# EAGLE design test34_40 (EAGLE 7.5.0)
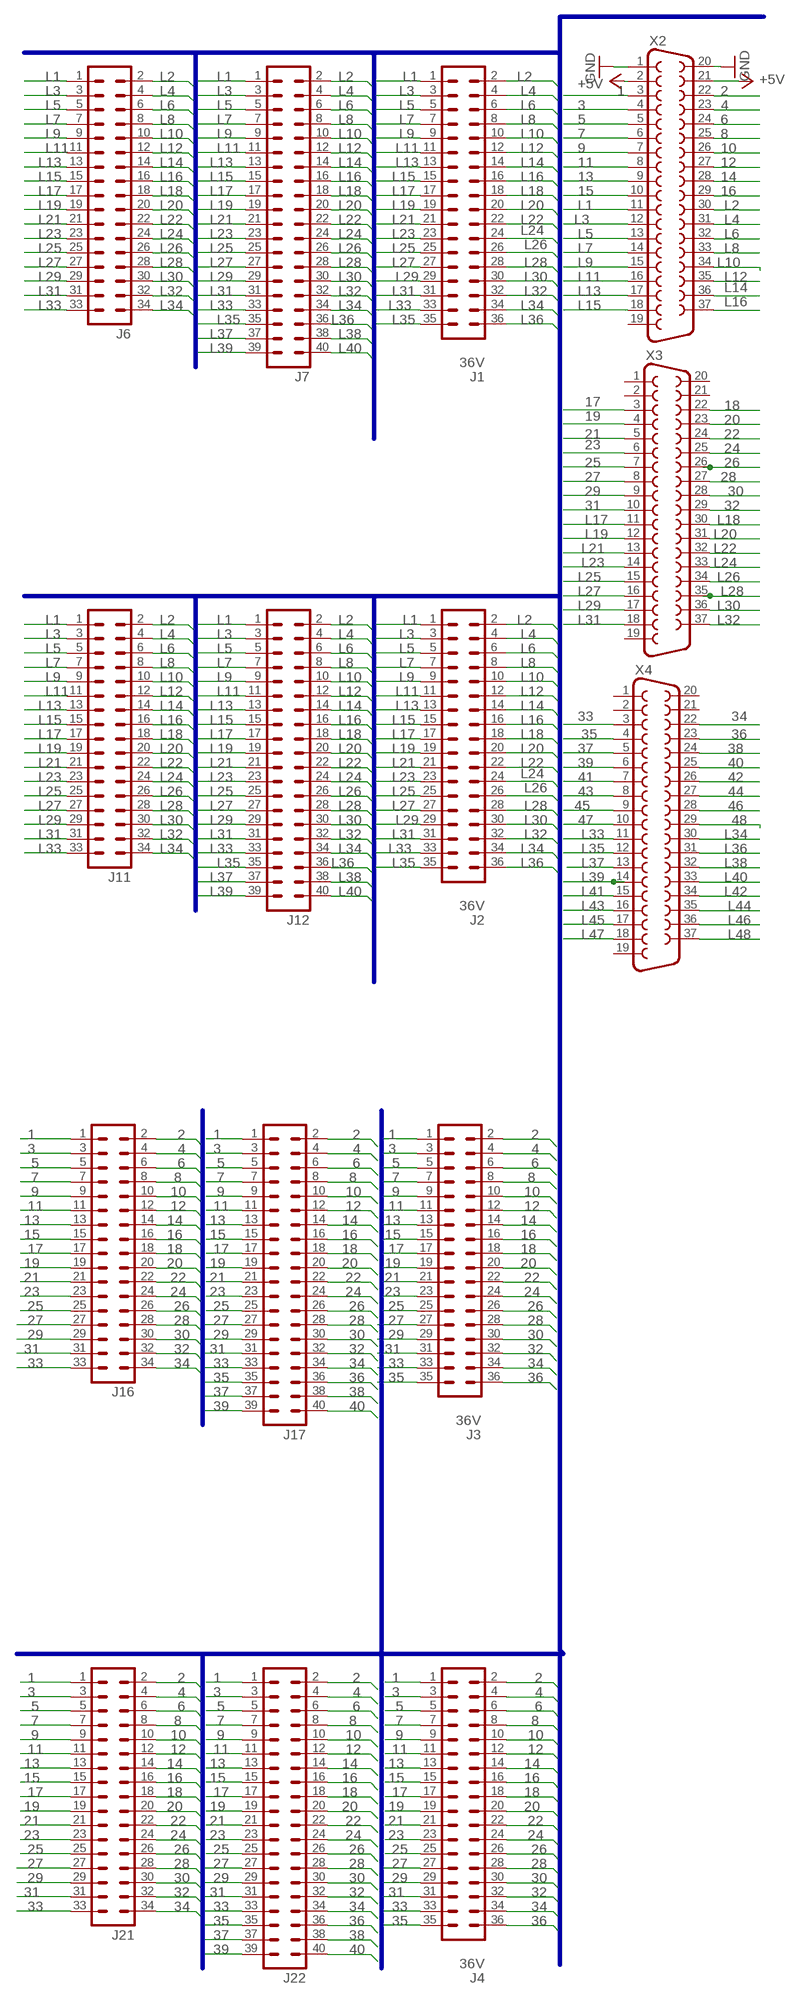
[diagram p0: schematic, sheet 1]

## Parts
J1  36V  [36V]
J2  36V  [36V]
J3  36V  [36V]
J4  36V  [36V]
J6  34V  [34V]
J7  40V  [40V]
J11  34V  [34V]
J12  40V  [40V]
J16  34V  [34V]
J17  40V  [40V]
J21  34V  [34V]
J22  40V  [40V]
X2  F37V  [F37V]
X3  F37V  [F37V]
X4  F37V  [F37V]

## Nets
1: J3.1 J4.1 J16.1 J17.1 J21.1 J22.1 X2.3
2: J3.2 J4.2 J16.2 J17.2 J21.2 J22.2 X2.22
3: J3.3 J4.3 J16.3 J17.3 J21.3 J22.3 X2.4
4: J3.4 J4.4 J16.4 J17.4 J21.4 J22.4 X2.23
5: J3.5 J4.5 J16.5 J17.5 J21.5 J22.5 X2.5
6: J3.6 J4.6 J16.6 J17.6 J21.6 J22.6 X2.24
7: J3.7 J4.7 J16.7 J17.7 J21.7 J22.7 X2.6
8: J3.8 J4.8 J16.8 J17.8 J21.8 J22.8 X2.25
9: J3.9 J4.9 J16.9 J17.9 J21.9 J22.9 X2.7
10: J3.10 J4.10 J16.10 J17.10 J21.10 J22.10 X2.26
11: J3.11 J4.11 J16.11 J17.11 J21.11 J22.11 X2.8
12: J3.12 J4.12 J16.12 J17.12 J21.12 J22.12 X2.27
13: J3.13 J4.13 J16.13 J17.13 J21.13 J22.13 X2.9
14: J3.14 J4.14 J16.14 J17.14 J21.14 J22.14 X2.28
15: J3.15 J4.15 J16.15 J17.15 J21.15 J22.15 X2.10
16: J3.16 J4.16 J16.16 J17.16 J21.16 J22.16 X2.29
17: J3.17 J4.17 J16.17 J17.17 J21.17 J22.17 X3.3
18: J3.18 J4.18 J16.18 J17.18 J21.18 J22.18 X3.22
19: J3.19 J4.19 J16.19 J17.19 J21.19 J22.19 X3.4
20: J3.20 J4.20 J16.20 J17.20 J21.20 J22.20 X3.23
21: J3.21 J4.21 J16.21 J17.21 J21.21 J22.21 X3.5
22: J3.22 J4.22 J16.22 J17.22 J21.22 J22.22 X3.24
23: J3.23 J4.23 J16.23 J17.23 J21.23 J22.23 X3.6
24: J3.24 J4.24 J16.24 J17.24 J21.24 J22.24 X3.25
25: J3.25 J4.25 J16.25 J17.25 J21.25 J22.25 X3.7
26: J3.26 J4.26 J16.26 J17.26 J21.26 J22.26 X3.26
27: J3.27 J4.27 J16.27 J17.27 J21.27 J22.27 X3.8
28: J3.28 J4.28 J16.28 J17.28 J21.28 J22.28 X3.27
29: J3.29 J4.29 J16.29 J17.29 J21.29 J22.29 X3.9
30: J3.30 J4.30 J16.30 J17.30 J21.30 J22.30 X3.28
31: J3.31 J4.31 J16.31 J17.31 J21.31 J22.31 X3.10
32: J3.32 J4.32 J16.32 J17.32 J21.32 J22.32 X3.29
33: J3.33 J4.33 J16.33 J17.33 J21.33 J22.33 X4.3
34: J3.34 J4.34 J16.34 J17.34 J21.34 J22.34 X4.22
35: J3.35 J4.35 J17.35 J22.35 X4.4
36: J3.36 J4.36 J17.36 J22.36 X4.23
37: J17.37 J22.37 X4.5
38: J17.38 J22.38 X4.24
39: J17.39 J22.39 X4.6
40: J17.40 J22.40 X4.25
41: X4.7
42: X4.26
43: X4.8
44: X4.27
45: X4.9
46: X4.28
47: X4.10
48: X4.29
+5V: X2.2 X2.21
GND: X2.1 X2.20
L1: J1.1 J2.1 J6.1 J7.1 J11.1 J12.1 X2.11
L2: J1.2 J2.2 J6.2 J7.2 J11.2 J12.2 X2.30
L3: J1.3 J2.3 J6.3 J7.3 J11.3 J12.3 X2.12
L4: J1.4 J2.4 J6.4 J7.4 J11.4 J12.4 X2.31
L5: J1.5 J2.5 J6.5 J7.5 J11.5 J12.5 X2.13
L6: J1.6 J2.6 J6.6 J7.6 J11.6 J12.6 X2.32
L7: J1.7 J2.7 J6.7 J7.7 J11.7 J12.7 X2.14
L8: J1.8 J2.8 J6.8 J7.8 J11.8 J12.8 X2.33
L9: J1.9 J2.9 J6.9 J7.9 J11.9 J12.9 X2.15
L10: J1.10 J2.10 J6.10 J7.10 J11.10 J12.10 X2.34
L11: J1.11 J2.11 J6.11 J7.11 J11.11 J12.11 X2.16
L12: J1.12 J2.12 J6.12 J7.12 J11.12 J12.12 X2.35
L13: J1.13 J2.13 J6.13 J7.13 J11.13 J12.13 X2.17
L14: J1.14 J2.14 J6.14 J7.14 J11.14 J12.14 X2.36
L15: J1.15 J2.15 J6.15 J7.15 J11.15 J12.15 X2.18
L16: J1.16 J2.16 J6.16 J7.16 J11.16 J12.16 X2.37
L17: J1.17 J2.17 J6.17 J7.17 J11.17 J12.17 X3.11
L18: J1.18 J2.18 J6.18 J7.18 J11.18 J12.18 X3.30
L19: J1.19 J2.19 J6.19 J7.19 J11.19 J12.19 X3.12
L20: J1.20 J2.20 J6.20 J7.20 J11.20 J12.20 X3.31
L21: J1.21 J2.21 J6.21 J7.21 J11.21 J12.21 X3.13
L22: J1.22 J2.22 J6.22 J7.22 J11.22 J12.22 X3.32
L23: J1.23 J2.23 J6.23 J7.23 J11.23 J12.23 X3.14
L24: J1.24 J2.24 J6.24 J7.24 J11.24 J12.24 X3.33
L25: J1.25 J2.25 J6.25 J7.25 J11.25 J12.25 X3.15
L26: J1.26 J2.26 J6.26 J7.26 J11.26 J12.26 X3.34
L27: J1.27 J2.27 J6.27 J7.27 J11.27 J12.27 X3.16
L28: J1.28 J2.28 J6.28 J7.28 J11.28 J12.28 X3.35
L29: J1.29 J2.29 J6.29 J7.29 J11.29 J12.29 X3.17
L30: J1.30 J2.30 J6.30 J7.30 J11.30 J12.30 X3.36
L31: J1.31 J2.31 J6.31 J7.31 J11.31 J12.31 X3.18
L32: J1.32 J2.32 J6.32 J7.32 J11.32 J12.32 X3.37
L33: J1.33 J2.33 J6.33 J7.33 J11.33 J12.33 X4.11
L34: J1.34 J2.34 J6.34 J7.34 J11.34 J12.34 X4.30
L35: J1.35 J2.35 J7.35 J12.35 X4.12
L36: J1.36 J2.36 J7.36 J12.36 X4.31
L37: J7.37 J12.37 X4.13
L38: J7.38 J12.38 X4.32
L39: J7.39 J12.39 X4.14
L40: J7.40 J12.40 X4.33
L41: X4.15
L42: X4.34
L43: X4.16
L44: X4.35
L45: X4.17
L46: X4.36
L47: X4.18
L48: X4.37
Unconnected: X2.19 X3.1 X3.2 X3.19 X3.20 X3.21 X4.1 X4.2 X4.19 X4.20 X4.21

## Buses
B$1

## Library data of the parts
J1-J4 = con-harting-v:36V
J6 J11 J16 J21 = con-harting-v:34V: CONNECTOR; OC_FARNELL: unknown; OC_NEWARK: unknown
J7 J12 J17 J22 = con-harting-v:40V: CONNECTOR; OC_FARNELL: unknown; OC_NEWARK: unknown
X2-X4 = con-subd:F37: SUB-D; OC_FARNELL: unknown; OC_NEWARK: unknown

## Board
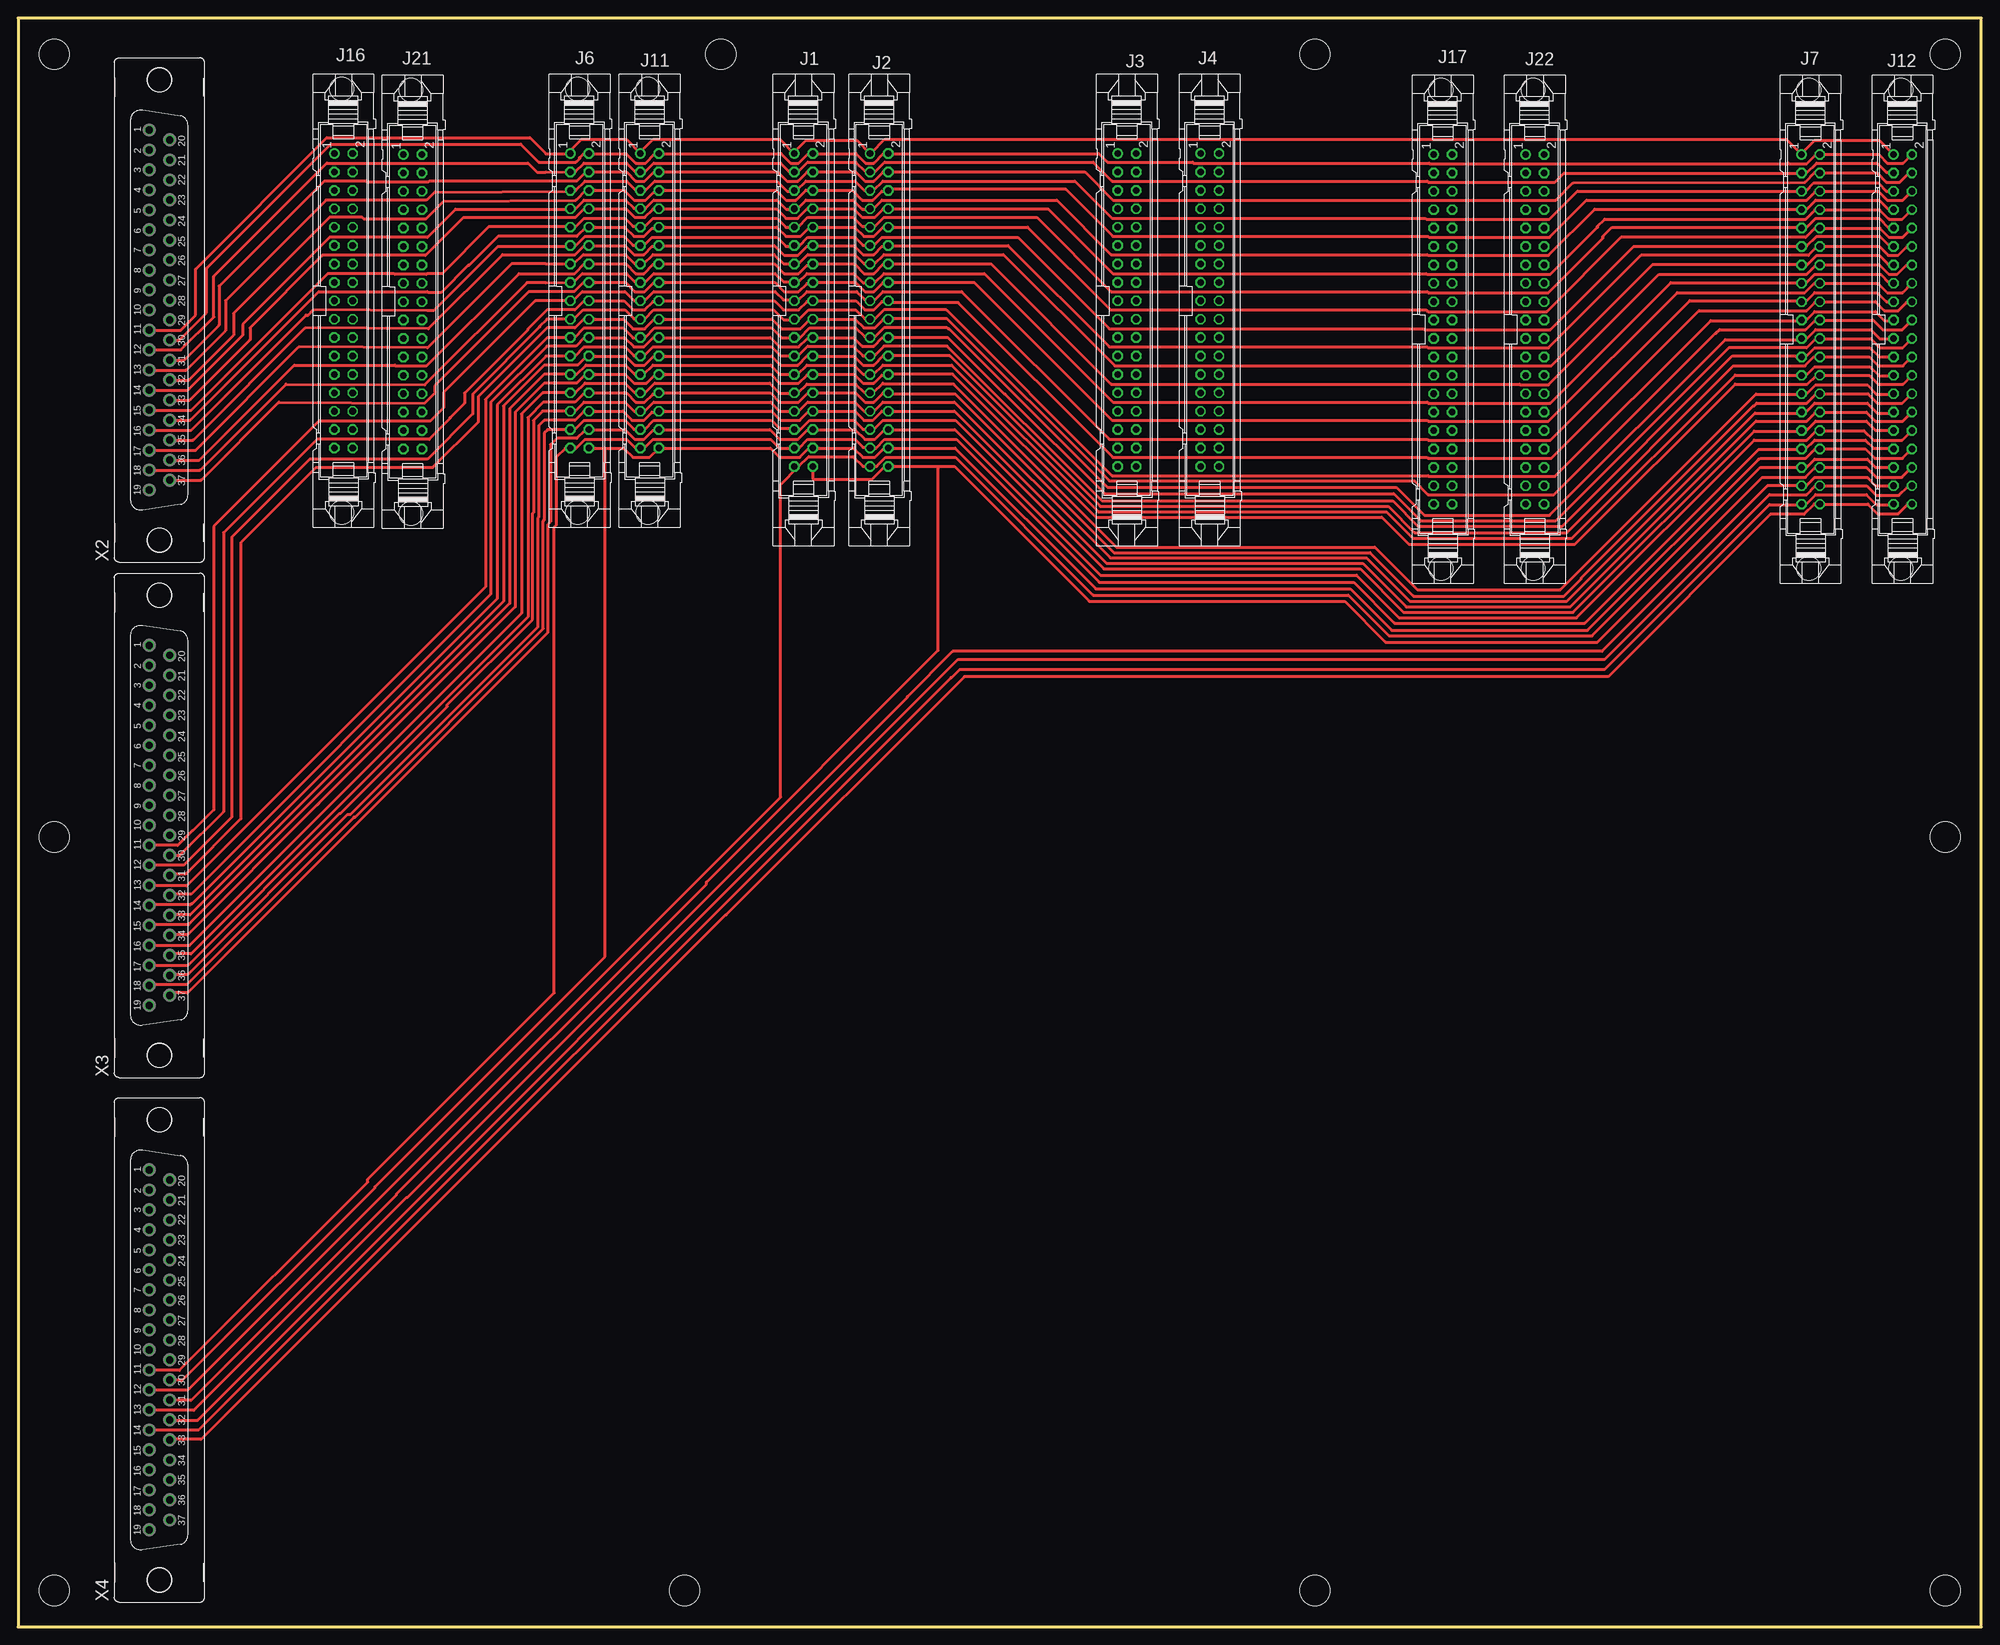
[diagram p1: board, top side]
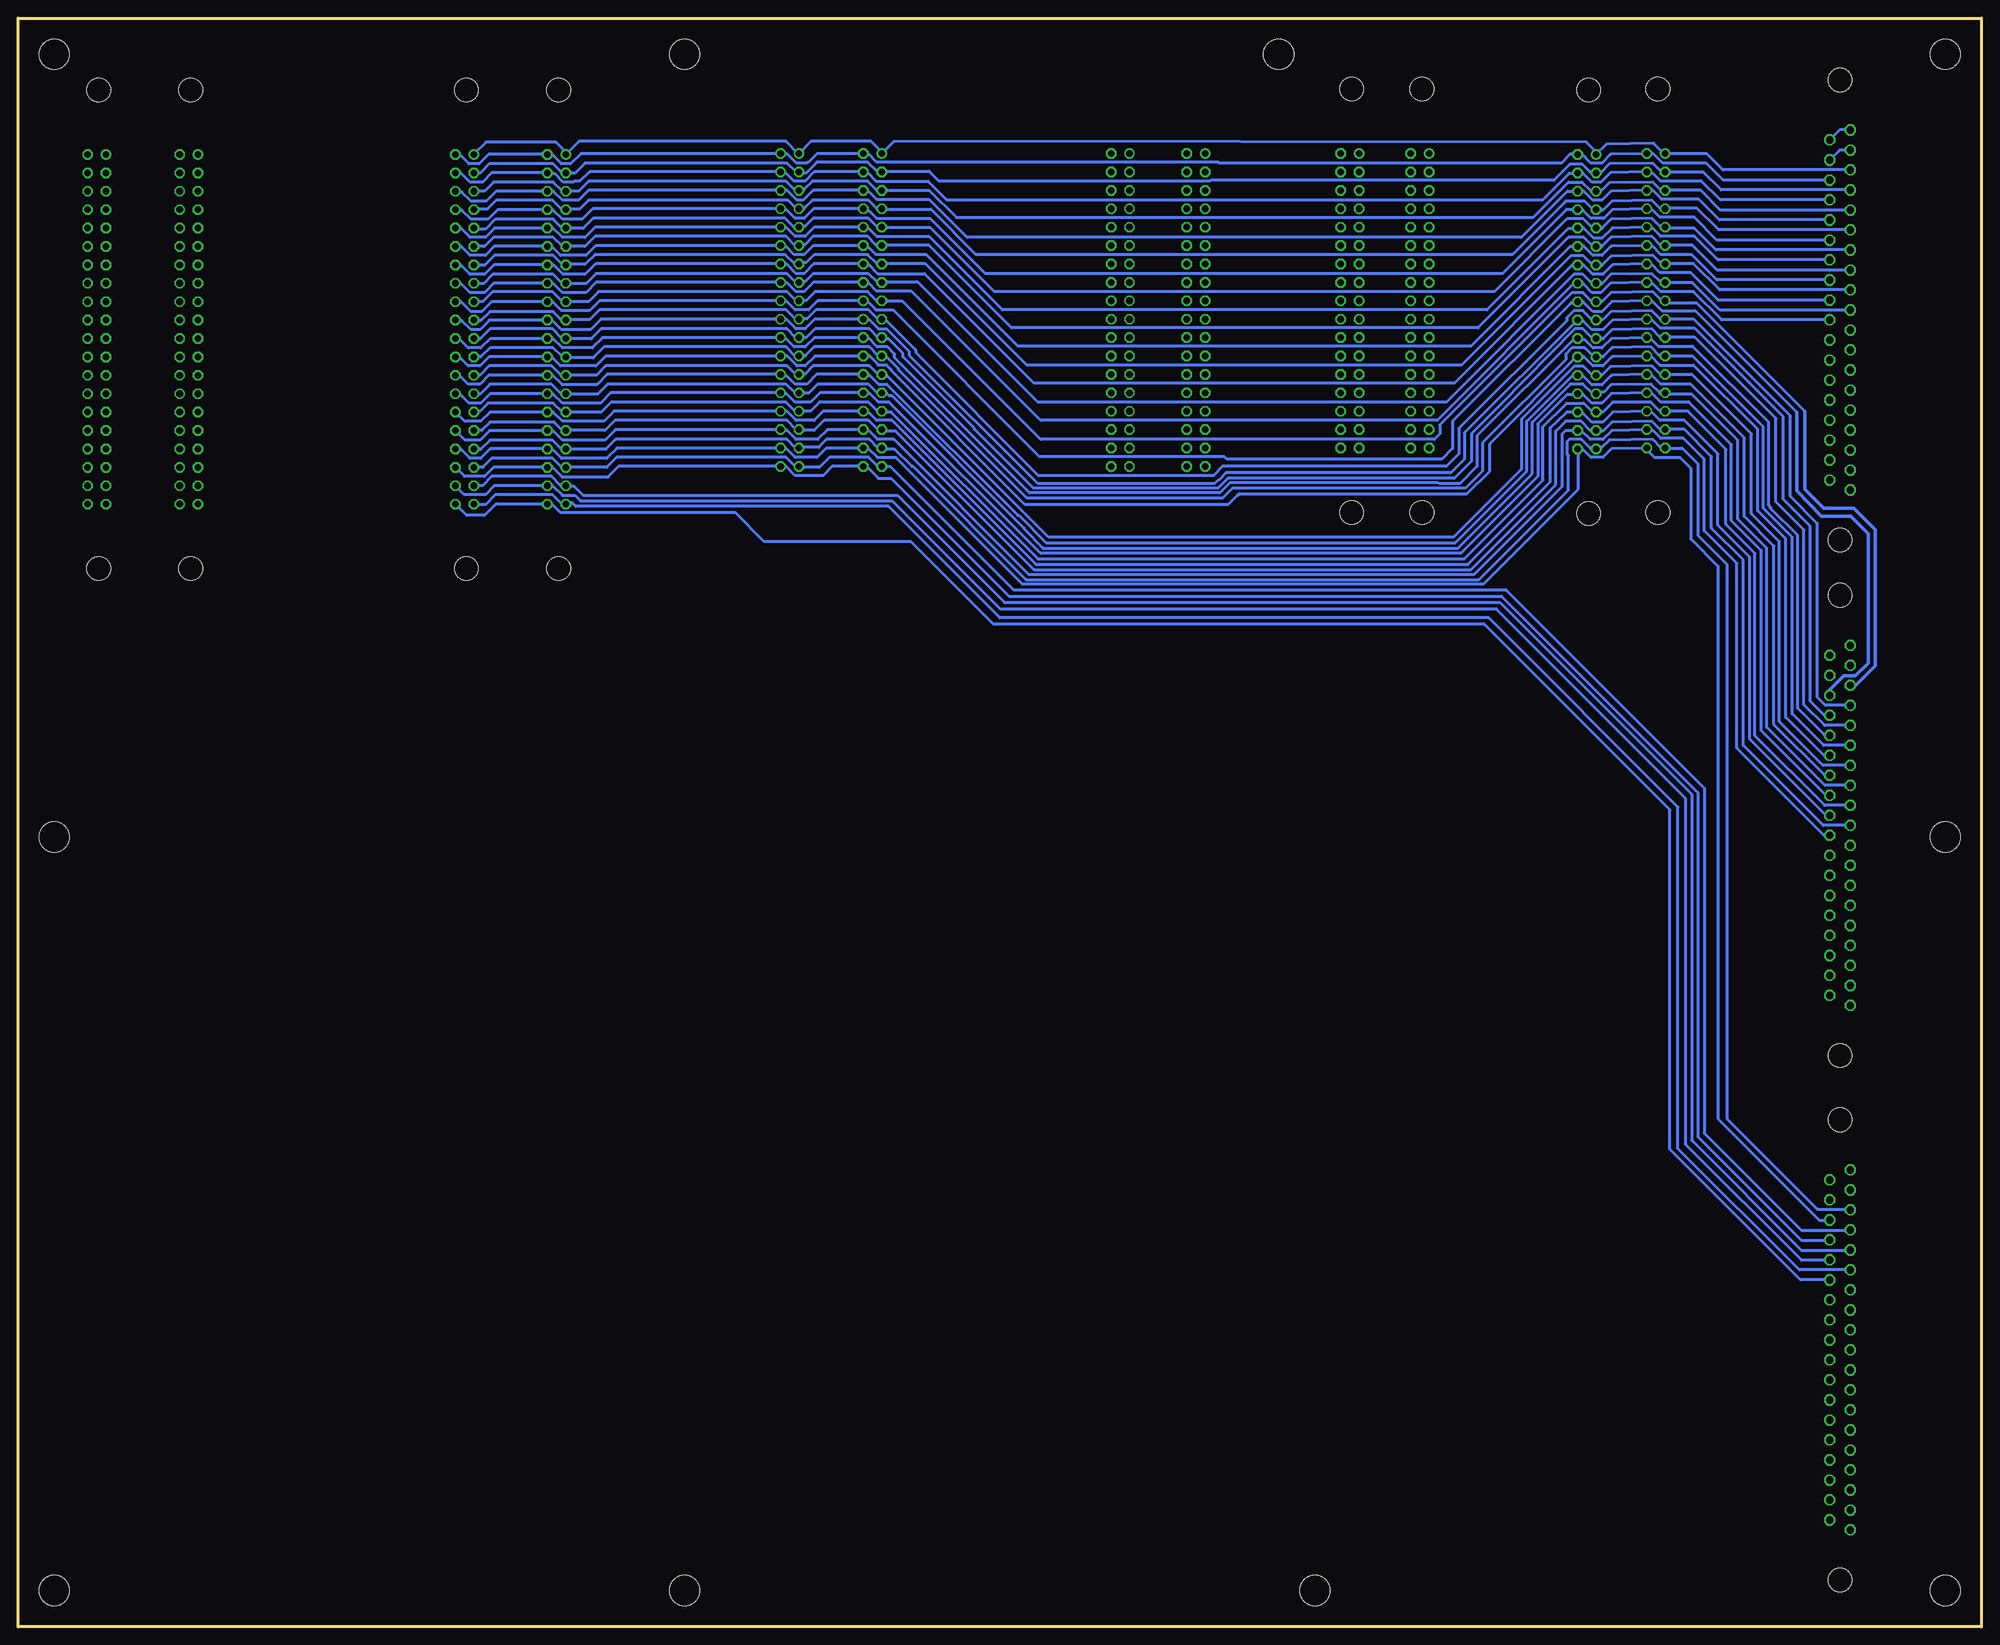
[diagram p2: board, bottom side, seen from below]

Size 271 x 222 mm. Coordinates in mm from the lower left corner, seen from the top.
Outline: 0,0 271,0 271,222 0,222 0,0
Copper layers (1*16): Top 0.035mm / dielectric 1.5mm / Bottom 0.035mm
Design rules "default": minimum track width 10mil, minimum drill 24mil, track to track 8mil, track to pad 8mil, pad to pad 8mil, via to via 8mil, smd to smd 8mil, copper to edge 40mil, drill to drill 8mil, minimum pad ring 10mil, minimum via ring 8mil, stop-mask expansion 4mil, vias tented up to drill 0mil, thermal gap 10mil
Holes 4.2 mm at 5,5 266,5 92,5 179,5 5,217 97,217 179,217 266,217 5,5 5,109 266,109

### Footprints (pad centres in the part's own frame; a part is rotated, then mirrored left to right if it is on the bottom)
36V = drill 0.914: 1 -20.32,0 | drill 0.914 octagon: 2 -20.32,2.54; 3 -17.78,0; 4 -17.78,2.54; 5 -15.24,0; 6 -15.24,2.54; 7 -12.7,0; 8 -12.7,2.54; 9 -10.16,0; 10 -10.16,2.54; 11 -7.62,0; 12 -7.62,2.54; 13 -5.08,0; 14 -5.08,2.54; 15 -2.54,0; 16 -2.54,2.54; 17 0,0; 18 0,2.54; 19 2.54,0; 20 2.54,2.54; 21 5.08,0; 22 5.08,2.54; 23 7.62,0; 24 7.62,2.54; 25 10.16,0; 26 10.16,2.54; 27 12.7,0; 28 12.7,2.54; 29 15.24,0; 30 15.24,2.54; 31 17.78,0; 32 17.78,2.54; 33 20.32,0; 34 20.32,2.54; 35 22.86,0; 36 22.86,2.54
34V = drill 0.914: 1 -20.32,-1.27 | drill 0.914 octagon: 2 -20.32,1.27; 3 -17.78,-1.27; 4 -17.78,1.27; 5 -15.24,-1.27; 6 -15.24,1.27; 7 -12.7,-1.27; 8 -12.7,1.27; 9 -10.16,-1.27; 10 -10.16,1.27; 11 -7.62,-1.27; 12 -7.62,1.27; 13 -5.08,-1.27; 14 -5.08,1.27; 15 -2.54,-1.27; 16 -2.54,1.27; 17 0,-1.27; 18 0,1.27; 19 2.54,-1.27; 20 2.54,1.27; 21 5.08,-1.27; 22 5.08,1.27; 23 7.62,-1.27; 24 7.62,1.27; 25 10.16,-1.27; 26 10.16,1.27; 27 12.7,-1.27; 28 12.7,1.27; 29 15.24,-1.27; 30 15.24,1.27; 31 17.78,-1.27; 32 17.78,1.27; 33 20.32,-1.27; 34 20.32,1.27 | hole 3.302: 29.21,-0.254; -29.21,-0.254
40V = drill 0.914: 1 -24.13,-1.27 | drill 0.914 octagon: 2 -24.13,1.27; 3 -21.59,-1.27; 4 -21.59,1.27; 5 -19.05,-1.27; 6 -19.05,1.27; 7 -16.51,-1.27; 8 -16.51,1.27; 9 -13.97,-1.27; 10 -13.97,1.27; 11 -11.43,-1.27; 12 -11.43,1.27; 13 -8.89,-1.27; 14 -8.89,1.27; 15 -6.35,-1.27; 16 -6.35,1.27; 17 -3.81,-1.27; 18 -3.81,1.27; 19 -1.27,-1.27; 20 -1.27,1.27; 21 1.27,-1.27; 22 1.27,1.27; 23 3.81,-1.27; 24 3.81,1.27; 25 6.35,-1.27; 26 6.35,1.27; 27 8.89,-1.27; 28 8.89,1.27; 29 11.43,-1.27; 30 11.43,1.27; 31 13.97,-1.27; 32 13.97,1.27; 33 16.51,-1.27; 34 16.51,1.27; 35 19.05,-1.27; 36 19.05,1.27; 37 21.59,-1.27; 38 21.59,1.27; 39 24.13,-1.27; 40 24.13,1.27 | hole 3.302: 33.02,-0.254; -33.02,-0.254
F37V = drill 1.016 octagon: 1 24.841,1.422; 2 22.073,1.422; 3 19.329,1.422; 4 16.561,1.422; 5 13.792,1.422; 6 11.049,1.422; 7 8.28,1.422; 8 5.512,1.422; 9 2.769,1.422; 10 0,1.422; 11 -2.769,1.422; 12 -5.512,1.422; 13 -8.28,1.422; 14 -11.049,1.422; 15 -13.818,1.422; 16 -16.561,1.422; 17 -19.329,1.422; 18 -22.098,1.422; 19 -24.841,1.422; 20 23.47,-1.422; 21 20.701,-1.422; 22 17.932,-1.422; 23 15.189,-1.422; 24 12.421,-1.422; 25 9.652,-1.422; 26 6.909,-1.422; 27 4.14,-1.422; 28 1.372,-1.422; 29 -1.372,-1.422; 30 -4.14,-1.422; 31 -6.909,-1.422; 32 -9.677,-1.422; 33 -12.421,-1.422; 34 -15.189,-1.422; 35 -17.958,-1.422; 36 -20.701,-1.422; 37 -23.47,-1.422 | hole 3.302: 31.75,0; -31.75,0

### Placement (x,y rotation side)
J1  107.14,182.99 270 top
J2  117.59,182.99 270 top
J3  151.78,182.99 270 top
J4  163.22,182.99 270 top
J6  77.5,182.99 270 top
J7  247.43,179.06 270 top
J11  87.17,182.99 270 top
J12  260.13,179.06 270 top
J16  44.91,182.99 270 top
J17  196.66,179.06 270 top
J21  54.47,182.87 270 top
J22  209.36,179.06 270 top
X2  19.51,181.72 90 top
X3  19.51,110.6 90 top
X4  19.51,38.21 90 top

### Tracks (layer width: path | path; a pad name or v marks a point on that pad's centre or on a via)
1
  Bottom 0.406: X2.3 35.67,201.05 37.88,203.25 43.58,203.25 J16.1 43.81,203.31 45.25,204.75 51.76,204.62 J21.1 53.2,203.57 54.5,204.88 150.09,205 J3.1 151.78,203.53 153.25,205 161.53,205 J4.1 163.31,203.31 165,205 193.57,205 J17.1 195.39,203.51 196.75,204.88 206.4,204.88 J22.1
2
  Bottom 0.406: X2.22 35.65,199.65 38,202 44,202 45.25,203.25 46.12,203.25 J16.2 51.19,203.19 52.38,202 53.88,202 55.12,203.25 55.67,203.25 J21.2 55.8,203.25 56.75,203.25 58,202 105.25,202 105.38,202.12 152.5,202.12 153.62,203.25 154.26,203.25 J3.2 160.69,203.31 161.88,202.12 162,202.12 162.12,202 163.57,202 164.88,203.31 J4.2 193.31,203.31 194.75,201.88 196,201.88 197.25,203.12 197.87,203.12 J17.2 206.06,203.19 207.38,201.88 208.75,201.88 210,203.12 210.57,203.12 J22.2
3
  Bottom 0.406: X2.4 35.91,198.28 38.38,200.75 43.62,200.75 J16.3 44.15,200.77 45.38,202 51.38,201.88 52.62,200.62 53.17,200.62 J21.3 53.9,200.65 55.12,201.88 56.75,201.88 59,199.62 106.38,199.62 106.5,199.5 143.88,199.5 145.25,200.88 151.68,200.88 J3.3 152.4,200.77 153.75,202.12 160.75,202.12 162.25,200.62 163.07,200.62 J4.3 163.65,200.77 164.88,202 192.75,202 194.12,200.62 195.37,200.62 J17.3 195.9,200.65 197.12,201.88 206,201.88 207.25,200.62 208.07,200.62 J22.3
4
  Bottom 0.406: X2.23 36.03,196.91 38.62,199.5 44.25,199.5 45.5,200.75 46.16,200.75 J16.4 51.23,200.65 52.5,199.38 53.75,199.38 55,200.62 55.72,200.62 J21.4 55.76,200.62 56.88,200.62 60.62,196.88 142.75,196.88 145.38,199.5 152.56,199.5 153.82,200.77 J3.4 161.1,200.77 162.38,199.5 163.88,199.5 165,200.62 165.61,200.62 J4.4 192.1,200.77 193.5,199.5 194.25,199.5 194.38,199.38 195.75,199.38 196.88,200.5 197.78,200.5 J17.4 205.6,200.65 206.88,199.38 208.62,199.38 209.88,200.62 210.61,200.62 J22.4
5
  Bottom 0.406: X2.5 36.01,195.51 38.75,198.25 43.62,198.25 J16.5 44.23,198.23 45.38,199.38 51.38,199.25 52.38,198.25 53.05,198.25 J21.5 53.85,198.1 55.12,199.38 57,199.38 61.88,194.5 141.5,194.5 145.23,198.23 J3.5 152.48,198.23 153.75,199.5 161.38,199.5 162.5,198.38 163.07,198.38 J4.5 163.73,198.23 165,199.5 192.25,199.5 193.62,198.12 195.37,198.12 J17.5 195.85,198.1 197.12,199.38 205.38,199.38 206.62,198.12 208.07,198.12 J22.5
6
  Bottom 0.406: X2.24 36.14,194.14 39,197 44.12,197 45.5,198.38 46.03,198.38 J16.6 51.15,198.1 52.38,196.88 53.62,196.88 54.88,198.12 55.72,198.12 J21.6 55.76,198.12 57.12,198.12 63.5,191.75 140,191.75 145.25,197 152.5,197 153.73,198.23 J3.6 161.27,198.23 162.62,196.88 163.5,196.88 164.88,198.25 165.74,198.25 J4.6 192.27,198.23 193.62,196.88 195.88,196.88 197.12,198.12 197.91,198.12 J17.6 205.02,198.1 206.38,196.75 208.5,196.75 209.75,198 210.53,198 J22.6
7
  Bottom 0.406: X2.6 36.27,192.77 39.25,195.75 43.58,195.75 J16.7 44.31,195.69 45.5,196.88 51,196.75 52.25,195.5 53.13,195.5 J21.7 53.56,195.56 54.75,196.75 57.38,196.75 64.75,189.38 138.75,189.38 145,195.62 151.72,195.62 J3.7 152.44,195.69 153.62,196.88 161.38,196.88 162.5,195.75 163.16,195.75 J4.7 163.56,195.69 164.75,196.88 192.25,196.88 193.5,195.62 195.33,195.62 J17.7 195.94,195.56 197.25,196.88 205,196.88 206.25,195.62 208.03,195.62 J22.7
8
  Bottom 0.406: X2.25 36.5,191.37 39.62,194.5 44.38,194.5 45.38,195.5 45.99,195.5 J16.8 50.94,195.56 52.12,194.38 53.88,194.38 55,195.5 55.67,195.5 J21.8 55.8,195.62 57.25,195.62 66.12,186.75 137.5,186.75 145.12,194.38 152.5,194.38 153.5,195.38 154.01,195.38 J3.8 161.19,195.69 162.5,194.38 163.75,194.38 165,195.62 165.69,195.62 J4.8 191.69,195.69 193.12,194.25 195.88,194.25 197.12,195.5 197.87,195.5 J17.8 204.81,195.56 206.12,194.25 208.5,194.25 209.75,195.5 210.56,195.5 J22.8
9
  Bottom 0.406: X2.7 36.62,190 39.62,193 43.49,193 J16.9 44.27,193.15 45.5,194.38 51.12,194.25 52.38,193 53.17,193 J21.9 53.65,193.03 55,194.38 57.12,194.38 67.25,184.25 136.25,184.25 145.12,193.12 151.76,193.12 J3.9 152.4,193.15 153.62,194.38 161.25,194.38 162.38,193.25 163.12,193.25 J4.9 163.9,193.15 165.12,194.38 191.62,194.38 193,193 195.37,193 J17.9 195.9,193.03 197.12,194.25 205.12,194.25 206.5,192.88 207.94,192.88 J22.9
10
  Bottom 0.406: X2.26 36.38,188.63 39.62,191.88 44.25,191.88 45.5,193.12 46.16,193.12 J16.10 50.98,193.03 52.38,191.62 53.5,191.62 54.88,193 55.71,193 J21.10 55.76,193 57,193 68.25,181.75 135.12,181.75 145.25,191.88 152.5,191.88 153.62,193 154.18,193 J3.10 161.1,193.15 162.38,191.88 163.75,191.88 165,193.12 165.73,193.12 J4.10 191.35,193.15 192.75,191.75 195.88,191.75 197.12,193 197.91,193 J17.10 205.22,193.03 206.5,191.75 208.62,191.75 209.88,193 210.6,193 J22.10
11
  Bottom 0.406: X2.8 36.48,187.23 39.88,190.62 43.62,190.62 J16.11 44.23,190.61 45.5,191.88 51.12,191.75 52.38,190.5 53.18,190.5 J21.11 53.61,190.49 54.88,191.75 57,191.75 69.5,179.25 133.88,179.25 145.25,190.62 151.77,190.62 J3.11 152.49,190.61 153.75,191.88 161.25,191.88 162.38,190.75 163.07,190.75 J4.11 163.74,190.61 165,191.88 191.38,191.88 192.75,190.5 195.38,190.5 J17.11 195.86,190.49 197.12,191.75 205.38,191.75 206.62,190.5 208.07,190.5 J22.11
12
  Bottom 0.406: X2.27 36.48,185.86 40,189.38 44.25,189.38 45.5,190.62 46.16,190.62 J16.12 51.14,190.49 52.38,189.25 53.62,189.25 54.88,190.5 55.72,190.5 J21.12 56.75,190.5 70.5,176.75 133,176.75 145.62,189.38 152.59,189.38 153.82,190.61 J3.12 161.26,190.61 162.5,189.38 163.88,189.38 165.12,190.62 165.74,190.62 J4.12 191.26,190.61 192.62,189.25 196.12,189.25 197.38,190.5 197.91,190.5 J17.12 205.26,190.49 206.5,189.25 208.62,189.25 209.88,190.5 210.62,190.5 J22.12
13
  Bottom 0.406: X2.9 36.11,184.49 39.75,188.12 43.59,188.12 J16.13 44.2,188.07 45.38,189.25 51.12,189.12 52.38,187.88 53.12,187.88 J21.13 53.7,187.94 55,189.25 56.62,189.25 71.75,174.12 131.75,174.12 145.75,188.12 151.73,188.12 J3.13 | 151.72,188 J3.13 | J3.13 152.44,188.07 153.75,189.38 161.12,189.38 162.25,188.25 163.03,188.25 J4.13 163.82,188.07 165.12,189.38 191.38,189.38 192.75,188 195.34,188 J17.13 195.82,187.94 197.12,189.25 205.25,189.25 206.62,187.88 208.02,187.88 J22.13
14
  Bottom 0.406: X2.28 36.34,183.09 40.12,186.88 44.38,186.88 45.5,188 46.11,188 J16.14 50.93,187.94 52.25,186.62 53.62,186.62 54.88,187.88 55.66,187.88 J21.14 55.79,188 56.38,188 72.75,171.62 130.75,171.62 145.88,186.75 152.38,186.75 153.7,188.07 J3.14 161.18,188.07 162.5,186.75 163.62,186.75 164.88,188 165.69,188 J4.14 191.31,188.07 192.75,186.62 195.75,186.62 197,187.88 197.86,187.88 J17.14 205.31,187.94 206.62,186.62 208.62,186.62 209.88,187.88 210.56,187.88 J22.14
15
  Bottom 0.406: X2.10 36.09,181.72 39.88,185.5 43.61,185.5 J16.15 44.28,185.53 45.5,186.75 51.12,186.62 52.38,185.38 53.16,185.38 J21.15 53.78,185.41 55,186.62 56.25,186.62 73.88,169 130.25,169 146.88,185.62 151.69,185.62 J3.15 152.41,185.53 153.62,186.75 161.25,186.75 162.38,185.62 163.12,185.62 J4.15 163.66,185.53 164.88,186.75 191.25,186.75 192.62,185.38 195.36,185.38 J17.15 195.91,185.41 197.12,186.62 205.5,186.62 206.75,185.38 208.06,185.38 J22.15
16
  Bottom 0.406: X2.29 35.85,180.35 39.75,184.25 44.25,184.25 45.5,185.5 46.15,185.5 J16.16 51.22,185.41 52.5,184.12 53.75,184.12 54.88,185.25 55.58,185.25 J21.16 55.89,185.25 56.38,185.25 75.12,166.5 129.88,166.5 147.75,184.38 152.54,184.38 153.7,185.53 J3.16 161.22,185.53 162.5,184.25 163.62,184.25 164.88,185.5 165.72,185.5 J4.16 191.22,185.53 192.62,184.12 195.88,184.12 197.25,185.5 197.84,185.5 J17.16 205.34,185.41 206.62,184.12 208.62,184.12 209.88,185.38 210.6,185.38 J22.16
17
  Bottom 0.406: J16.17 44.12,182.99 45.38,184.25 51.12,184.12 52.38,182.88 53.19,182.88 J21.17 53.74,182.87 55,184.12 56.5,184.12 74.75,165.88 74.75,164.62 75.5,163.88 129.88,163.88 148.99,182.99 J3.17 | 43.4,182.75 39.38,182.75 24.38,167.75 | J3.17 | J3.17 152.49,182.99 153.75,184.25 161,184.25 162.25,183 163.21,183 J4.17 163.62,182.99 164.88,184.25 190.88,184.25 192.25,182.88 J17.17 195.87,182.87 197.25,184.25 205.5,184.25 206.88,182.88 J22.17
  Bottom 0.51: X3.3 17.32,129.93 14.62,132.62 14.62,151.38 17.62,154.38 21.75,154.38 24.38,157 24.38,167.75 | 43.4,182.75 J16.17
18
  Bottom 0.406: 25.5,167.62 39.5,181.62 44.12,181.62 45.5,183 J16.18 51.01,182.87 52.38,181.5 53.62,181.5 55,182.88 55.73,182.88 J21.18 55.85,182.75 56.62,182.75 73,166.38 73,162.62 74.5,161.12 104.12,161.12 104.5,161.5 130,161.5 150.25,181.75 152.59,181.75 153.82,182.99 J3.18 160.63,182.99 161.88,181.75 163.75,181.75 165,183 J4.18 190.76,182.99 192.12,181.62 196,181.62 197.25,182.88 J17.18 205.63,182.87 207,181.5 208.5,181.5 209.88,182.88 J22.18
  Bottom 0.51: X3.22 20.93,129.32 19,131.25 17.38,131.25 15.62,133 15.62,150.88 18,153.25 22.12,153.25 25.5,156.75 25.5,167.62
19
  Bottom 0.406: X3.4 21.54,127.16 22.62,128.25 22.62,152.25 26.38,156 26.38,167.12 39.75,180.5 43.59,180.5 J16.19 44.33,180.45 45.5,181.62 51.12,181.5 52.25,180.38 53.15,180.38 J21.19 53.7,180.32 55,181.62 56.25,181.62 57.25,180.62 57.25,180.25 72.12,165.38 72.12,161.88 73.88,160.12 104.75,160.12 106,158.88 130.12,158.88 147.12,175.88 147.12,176.25 151.25,180.38 151.71,180.38 J3.19 152.32,180.45 153.62,181.75 160.88,181.75 162.12,180.5 163.16,180.5 J4.19 163.7,180.45 165,181.75 190.75,181.75 192.12,180.38 195.34,180.38 J17.19 195.95,180.32 197.12,181.5 205.88,181.5 207.12,180.25 208.01,180.25 J22.19
20
  Bottom 0.406: X3.23 21.66,125.79 23.62,127.75 23.62,151.88 27.38,155.62 27.38,167 39.62,179.25 44.38,179.25 45.5,180.38 46.1,180.38 J16.20 50.92,180.32 52.25,179 53.75,179 55,180.25 55.66,180.25 J21.20 55.8,180.32 71.38,164.75 71.38,161.12 73.25,159.25 104.25,159.25 105.25,158.25 105.38,158.25 105.88,157.75 130.25,157.75 148,175.5 148,176 151.12,179.12 152.25,179.12 153.5,180.38 154.25,180.38 J3.20 161.05,180.45 162.38,179.12 163.62,179.12 164.88,180.38 165.68,180.38 J4.20 190.55,180.45 192,179 196,179 197.25,180.25 197.85,180.25 J17.20 205.93,180.32 207.25,179 208.5,179 209.75,180.25 210.56,180.25 J22.20
21
  Bottom 0.406: X3.5 21.64,124.39 24.5,127.25 24.5,151.38 28.38,155.25 28.38,166.75 39.62,178 43.55,178 J16.21 44.28,177.91 45.5,179.12 51,179 52.25,177.75 53.16,177.75 J21.21 53.66,177.78 55,179.12 56.12,179.12 66.38,168.62 70.38,164.62 70.38,160.88 72.75,158.5 104,158.5 105.38,157.12 130.88,157.12 139,165.25 139,165.38 148.88,175.25 148.88,175.75 150.88,177.75 151.62,177.75 J3.21 | 151.69,178 J3.21 | J3.21 152.28,177.91 153.5,179.12 161,179.12 162.25,177.88 163.18,177.88 J4.21 163.66,177.91 164.88,179.12 190.5,179.12 191.88,177.75 195.35,177.75 J17.21 195.91,177.78 197.25,179.12 205.88,179.12 207.25,177.75 208.06,177.75 J22.21
22
  Bottom 0.406: X3.24 21.65,123.02 25.38,126.75 25.38,150.62 29.12,154.38 29.12,154.5 29.38,154.75 29.38,166.25 39.88,176.75 44.62,176.75 45.62,177.75 46.02,177.75 J16.22 51.09,177.78 52.38,176.5 53.62,176.5 54.75,177.62 55.58,177.62 J21.22 56.22,177.78 69.62,164.38 69.62,160.12 72,157.75 74.88,157.75 75,157.88 103.75,157.88 105.12,156.5 131.38,156.5 150,175.12 150,175.62 151,176.62 152.41,176.62 152.41,176.66 153.62,177.88 154.29,177.88 J3.22 161.09,177.91 162.38,176.62 163.88,176.62 165.12,177.88 165.72,177.88 J4.22 190.34,177.91 191.75,176.5 195.88,176.5 197.12,177.75 197.9,177.75 J17.22 205.84,177.78 207.12,176.5 208.88,176.5 210.12,177.75 210.59,177.75 J22.22
23
  Bottom 0.406: X3.6 21.77,121.65 26.12,126 26.12,150.38 30.12,154.38 30.12,165.62 39.88,175.38 J16.23 44.37,175.37 45.62,176.62 51,176.5 52.25,175.25 J21.23 53.49,175.25 54.75,176.5 56.5,176.5 57.38,175.62 57.38,174.88 68.88,163.38 68.88,159.5 71.25,157.12 103.38,157.12 104.75,155.75 131.75,155.75 149.5,173.5 149.5,173.62 151.12,175.25 151.66,175.25 J3.23 | J3.23 | J3.23 152.25,175.37 153.5,176.62 161.12,176.62 162.38,175.38 J4.23 163.75,175.37 165,176.62 190.12,176.62 191.62,175.12 195.27,175.12 J17.23 195.87,175.25 197.12,176.5 205.88,176.5 207.12,175.25 J22.23
24
  Bottom 0.406: X3.25 21.75,120.25 27,125.5 27,150.12 30.88,154 30.88,165.25 39.75,174.12 44.38,174.12 45.62,175.38 J16.24 51.01,175.25 52.25,174 53.62,174 54.88,175.25 J21.24 55.88,175.25 67.88,163.25 67.88,159.5 71,156.38 102.38,156.38 102.5,156.25 102.62,156.25 104,154.88 132,154.88 150.5,173.38 150.5,173.5 151.12,174.12 152.33,174.12 152.33,174.21 153.5,175.38 J3.24 161,175.37 162.38,174 163.5,174 164.88,175.38 J4.24 189.88,175.37 191.25,174 196.12,174 197.25,175.12 197.81,175.12 J17.24 206,175.25 207.25,174 208.88,174 210.12,175.25 J22.24
25
  Bottom 0.406: X3.7 21.88,118.88 27.88,124.88 27.88,149.75 31.75,153.62 31.75,164.62 40,172.88 43.59,172.88 J16.25 44.33,172.83 45.5,174 51.25,173.88 52.38,172.75 53.15,172.75 J21.25 53.7,172.71 55,174 56.12,174 63.5,166.62 63.5,159.75 72.88,150.38 128.75,150.38 151.12,172.75 151.71,172.75 J3.25 | 151.74,172.88 J3.25 | J3.25 152.33,172.83 153.5,174 161.25,174 162.38,172.88 163.17,172.88 J4.25 163.71,172.83 164.88,174 189.88,174 191.12,172.75 195.34,172.75 J17.25 196.08,172.71 197.38,174 206,174 207.25,172.75 208.04,172.75 J22.25
26
  Bottom 0.406: X3.26 21.63,117.51 28.62,124.5 28.62,149.12 32.75,153.25 32.75,164.12 40.12,171.5 44.25,171.5 45.62,172.88 46.13,172.88 J16.26 51.05,172.71 52.38,171.38 53.75,171.38 55,172.62 55.66,172.62 J21.26 55.78,172.75 56.38,172.75 62.75,166.38 62.75,159.5 72.62,149.62 129.12,149.62 132.88,153.38 132.99,153.38 151.11,171.5 152.25,171.5 153.58,172.83 J3.26 160.79,172.83 162.12,171.5 163.75,171.5 165,172.75 165.68,172.75 J4.26 189.67,172.83 191,171.5 191.12,171.5 191.25,171.38 195.88,171.38 197.25,172.75 197.88,172.75 J17.26 206.04,172.71 207.25,171.5 208.88,171.5 210.12,172.75 210.59,172.75 J22.26
27
  Bottom 0.406: X3.8 21.61,116.11 29.62,124.12 29.62,148.88 33.62,152.88 33.62,163.75 40,170.12 43.48,170.12 J16.27 44.41,170.29 45.62,171.5 51.12,171.38 52.12,170.38 52.98,170.38 J21.27 53.66,170.16 55,171.5 56.75,171.5 62,166.25 62,159.12 72.25,148.88 129.5,148.88 132.12,151.5 132.12,151.62 150.38,169.88 150.75,169.88 151.12,170.25 151.25,170.12 151.62,170.12 J3.27 152.41,170.29 153.62,171.5 160.62,171.5 161.88,170.25 163.18,170.25 J4.27 163.79,170.29 165,171.5 189.62,171.5 191,170.12 195.35,170.12 J17.27 196.04,170.16 197.38,171.5 205.88,171.5 207.25,170.12 208.05,170.12 J22.27
28
  Bottom 0.406: X3.27 21.49,114.74 30.38,123.62 30.38,148.5 34.5,152.62 34.5,163.12 40.38,169 44.25,169 45.62,170.38 46.09,170.38 J16.28 51.09,170.16 52.38,168.88 53.75,168.88 55,170.12 55.7,170.12 J21.28 55.77,170.12 57.12,170.12 61.25,166 61.25,158.75 71.88,148.12 129.88,148.12 150.75,169 152.25,169 153.5,170.25 154.28,170.25 J3.28 160.34,170.29 161.62,169 163.75,169 165,170.25 165.72,170.25 J4.28 189.21,170.29 190.62,168.88 195.88,168.88 197.12,170.12 197.89,170.12 J17.28 205.84,170.16 207.12,168.88 208.75,168.88 210.12,170.25 210.54,170.25 J22.28
29
  Bottom 0.406: X3.9 21.62,113.37 31.25,123 31.25,148.12 35.25,152.12 35.25,162.5 40.5,167.75 J16.29 44.38,167.75 45.62,169 50.88,169 52.25,167.62 J21.29 53.62,167.62 54.88,168.88 57.25,168.88 60.5,165.62 60.5,158.25 71.38,147.38 130.25,147.38 150.5,167.62 151.66,167.62 J3.29 152.38,167.75 153.62,169 160.38,169 161.62,167.75 J4.29 163.75,167.75 165,169 189.12,169 190.5,167.62 J17.29 195.88,167.62 197.12,168.88 206.12,168.88 207.25,167.75 207.97,167.75 J22.29
30
  Bottom 0.406: X3.28 21.47,111.97 32,122.5 32,147.62 36.38,152 36.38,161.88 41,166.5 44.38,166.5 45.5,167.62 46.05,167.62 J16.30 50.88,167.62 52.25,166.25 53.75,166.25 55,167.5 55.61,167.5 J21.30 57.25,167.62 59.5,165.5 59.5,158 70.88,146.62 130.5,146.62 150.38,166.5 152.5,166.5 153.62,167.62 154.2,167.62 J3.30 159.88,167.75 161.12,166.5 163.62,166.5 164.88,167.75 J4.30 188.75,167.75 190.12,166.38 195.88,166.38 197.12,167.62 J17.30 205.88,167.62 207.12,166.38 209.38,166.38 J22.30
31
  Bottom 0.406: X3.10 21.85,110.6 32.88,121.62 32.88,147.25 37.25,151.62 37.25,161.5 41,165.25 43.6,165.25 J16.31 44.34,165.21 45.5,166.38 51,166.25 52.25,165 53.11,165 J21.31 53.96,165.09 55.25,166.38 57.38,166.38 58.75,165 58.75,157.62 70.5,145.88 130.75,145.88 149.88,165 151.57,165 J3.31 152.34,165.21 153.62,166.5 159.75,166.5 161.12,165.12 163.13,165.12 J4.31 163.59,165.21 164.88,166.5 188.62,166.5 190,165.12 195.35,165.12 J17.31 195.84,165.09 197,166.25 205.88,166.25 207,165.12 208.05,165.12 J22.31
32
  Bottom 0.406: X3.29 21.73,109.23 33.75,121.25 33.75,146.75 38.25,151.25 38.25,161.12 41.12,164 44.25,164 45.38,165.12 46.09,165.12 J16.32 51.04,165.09 52.25,163.88 54,163.88 55.12,165 55.65,165 J21.32 57.41,165.09 57.88,164.62 57.88,157.38 70,145.25 131.5,145.25 150.12,163.88 152.38,163.88 153.71,165.21 J3.32 159.29,165.21 160.62,163.88 163.62,163.88 164.88,165.12 165.67,165.12 J4.32 188.54,165.21 190,163.75 195.88,163.75 197.25,165.12 197.89,165.12 J17.32 205.91,165.09 207.25,163.75 209.29,163.75 J22.32
33
  Bottom 0.406: X4.3 18.17,57.62 22.62,57.62 35.12,70.12 35.12,146.62 39.12,150.62 39.12,160.5 41.3,162.67 J16.33 44.17,162.67 45.38,163.88 51.38,163.75 52.5,162.62 53.12,162.62 J21.33 53.92,162.54 55.25,163.88 56.88,163.88 57.12,163.62 57.12,161.75 57,161.62 57,156.88 69.38,144.5 131.88,144.5 147.5,160.12 147.62,160.12 150,162.5 151.62,162.5 J3.33 152.29,162.67 153.5,163.88 159.38,163.88 160.5,162.75 163.13,162.75 J4.33 163.67,162.67 164.88,163.88 188.5,163.88 189.88,162.5 195.34,162.5 J17.33 196.04,162.54 197.25,163.75 205.88,163.75 207.12,162.5 208.04,162.5 J22.33
34
  Bottom 0.406: X4.22 20.95,56.12 22.38,56.12 36.38,70.12 36.38,146.38 40.12,150.12 40.12,159.88 41.62,161.38 45.12,161.38 46.18,162.43 J16.34 51.08,162.54 52.25,161.38 53.88,161.38 55,162.5 55.69,162.5 J21.34 55.73,156.89 68.75,143.88 132.38,143.88 149.88,161.38 152.38,161.38 153.67,162.67 J3.34 159.46,162.67 160.75,161.38 163.75,161.38 165,162.62 165.71,162.62 J4.34 188.33,162.67 189.75,161.25 196,161.25 197.38,162.62 197.85,162.62 J17.34 205.83,162.54 207.12,161.25 208.62,161.25 209.88,162.5 210.59,162.5 J22.34
35
  Bottom 0.406: X4.4 18.11,54.75 24.88,54.75 38.25,68.12 38.25,115.75 65.62,143.12 133.62,143.12 150.63,160.13 J3.35 152.38,160.13 153.62,161.38 159,161.38 160.38,160 163.09,160 J4.35 163.75,160.13 165,161.38 188.38,161.38 189.75,160 J17.35 196,160 197.25,161.25 205.62,161.25 206.88,160 J22.35
36
  Bottom 0.406: X4.23 20.96,53.38 24.88,53.38 39.12,67.62 39.12,115.12 66.25,142.25 134.25,142.25 150.5,158.5 152.25,158.5 153.88,160.13 J3.36 158.62,160.13 159.88,158.88 163.75,158.88 165,160.12 J4.36 188.12,160.13 189.62,158.62 195.88,158.62 197.25,160 J17.36 205.37,160 206.62,158.75 209.38,158.75 J22.36
37
  Bottom 0.406: X4.5 24.88,52 40,67.12 40,114.88 66.5,141.38 134.88,141.38 149.62,156.12 193,156.12 194.34,157.47 J17.37 196.09,157.47 197.38,158.75 205.62,158.75 206.88,157.5 208.06,157.5 J22.37
38
  Bottom 0.406: X4.24 24.88,50.62 40.88,66.62 40.88,114.38 67,140.5 135.5,140.5 150.38,155.38 193.38,155.38 194.12,156.12 195.88,156.12 197.22,157.47 J17.38 205.28,157.47 206.5,156.25 209.41,156.25 J22.38
39
  Bottom 0.406: X4.6 25.13,49.26 41.88,66 41.88,113.12 68,139.25 135.5,139.25 150.88,154.62 194,154.62 194.5,155.12 195.19,155.12 J17.39 195.93,154.93 197.25,156.25 205.12,156.25 206.5,154.88 208.04,154.88 J22.39
40
  Bottom 0.406: X4.25 24.99,47.86 43,65.88 43,112.75 68.62,138.38 136.38,138.38 147.75,149.75 168,149.75 172,153.75 196.12,153.75 197.38,155 197.85,155 J17.40 205.07,154.93 206.62,153.38 209.08,153.38 J22.40
+5V
  Bottom 0.406: X2.2 19.56,203.79 X2.21
GND
  Bottom 0.406: X2.1 19.56,206.56 X2.20
L1
  Top 0.406: X2.11 22.45,178.95 24.5,181 24.5,187.38 42.62,205.5 70.66,205.5 70.66,205.47 72.88,203.25 76.17,203.25 J6.1 76.22,203.72 77.75,205.25 83.97,205.25 J11.1 85.91,203.53 87.62,205.25 105.2,205.25 J1.1 107.14,203.51 108.75,205.12 115.78,205.12 J2.1 117.81,203.31 117.81,203.44 119.62,205.25 244.09,205.25 J7.1 246.16,203.28 248,205.12 256.92,205.12 J12.1
L2
  Top 0.406: X2.30 22.2,177.58 26,181.38 26,187.5 43.12,204.62 69.38,204.62 71.88,202.12 77,202.12 77.5,202.62 77.5,202.75 78.06,203.31 J6.2 83.94,203.31 85.25,202 86.62,202 87.88,203.25 88.39,203.25 J11.2 105.31,203.31 106.62,202 107.75,202 109.06,203.31 J1.2 115.69,203.31 117,202 118.12,202 119.38,203.25 120.07,203.25 J2.2 149.19,203.31 150.38,202.12 162.12,202.12 162.25,202 194.75,202 194.88,201.88 244.25,201.88 244.38,202 244.5,201.88 246.88,201.88 248.12,203.12 248.64,203.12 J7.2 256.81,203.19 258,202 260.21,202 J12.2
L3
  Top 0.406: X2.12 22.46,176.21 27,180.75 27,186.38 42.62,202 70.38,202 71.62,200.75 72.83,200.75 J6.3 76.89,200.77 78.12,202 84,202 85.25,200.75 85.89,200.75 J11.3 86.52,200.77 87.75,202 105.25,202 106.38,200.88 107.03,200.88 J1.3 107.64,200.77 109,202.12 115.62,202.12 116.88,200.88 117.48,200.88 J2.3 118.27,200.77 119.62,202.12 148.38,202.12 151,199.5 194.5,199.5 194.62,199.38 212.12,199.38 213.38,200.62 246.14,200.62 J7.3 246.9,200.65 248.25,202 256.62,202 257.88,200.75 258.75,200.75 J12.3
L4
  Top 0.406: X2.31 22.94,174.81 27.75,179.62 27.75,185 42.25,199.5 48,199.5 48.12,199.38 56.62,199.38 56.75,199.5 77.12,199.5 78.39,200.77 J6.4 83.98,200.77 85.25,199.5 86.5,199.5 87.75,200.75 88.42,200.75 J11.4 104.86,200.77 106.12,199.5 107.62,199.5 108.88,200.75 109.66,200.75 J1.4 115.61,200.77 116.88,199.5 118.12,199.5 119.38,200.75 120.11,200.75 J2.4 147.23,200.77 151.12,196.88 212.25,196.88 214.62,199.25 246.68,199.38 247.95,200.65 J7.4 256.61,200.65 257.88,199.38 259.75,199.38 260.88,200.5 261.25,200.5 J12.4
L5
  Top 0.406: X2.13 23.19,173.44 28.62,178.88 28.62,183 42.5,196.88 56.38,196.88 57.5,198 76.12,198.12 J6.5 76.98,198.23 78.25,199.5 84,199.5 85.25,198.25 85.89,198.25 J11.5 86.61,198.23 87.88,199.5 104.75,199.5 106.12,198.12 107.03,198.12 J1.5 107.48,198.23 108.75,199.5 115.5,199.5 116.75,198.25 117.57,198.25 J2.5 118.11,198.23 119.38,199.5 145.88,199.5 151,194.38 194.25,194.38 194.38,194.25 211.38,194.25 215.25,198.12 246.14,198.12 J7.5 246.73,198.1 247.88,199.25 256.75,199.25 257.88,198.12 258.84,198.12 J12.5
L6
  Top 0.406: X2.32 23.54,172.04 29.75,178.25 29.75,181.25 43,194.5 47.5,194.5 47.75,194.25 56.25,194.25 58.75,196.75 77,196.87 78.36,198.23 J6.6 83.64,198.23 85,196.88 86.62,196.88 87.75,198 88.22,198 J11.6 104.64,198.23 106,196.88 107.38,196.88 108.75,198.25 109.66,198.25 J1.6 115.14,198.23 116.5,196.88 118,196.88 119.25,198.12 120.03,198.12 J2.6 120.28,198.38 144.62,198.38 151.12,191.88 194.62,191.88 194.75,191.75 211.38,191.75 216.5,196.88 246.88,196.88 248,198 248.59,198 J7.6 256.77,198.1 258,196.88 260.17,196.88 J12.6
L7
  Top 0.406: X2.14 23.42,170.67 31,178.25 31,179.75 43,191.75 56.5,191.75 60.38,195.62 76.16,195.62 J6.7 | 76.17,195.75 J6.7 | J6.7 76.94,195.69 78.12,196.88 83.88,196.88 85,195.75 85.84,195.75 J11.7 86.56,195.69 87.75,196.88 104.75,196.88 106,195.62 107.08,195.62 J1.7 107.56,195.69 108.75,196.88 115.25,196.88 116.5,195.62 117.53,195.62 J2.7 118.06,195.69 119.25,196.88 143.38,196.88 150.88,189.38 194.5,189.38 194.62,189.25 211.25,189.25 217.62,195.62 246.1,195.62 J7.7 246.81,195.56 248.12,196.88 256.88,196.88 258.12,195.62 258.8,195.62 J12.7
L8
  Top 0.406: X2.33 23.67,169.3 32,177.62 32,179.25 42,189.25 56.25,189.25 61.5,194.5 76.95,194.5 78.14,195.69 J6.8 83.94,195.69 85.12,194.5 86.5,194.5 87.62,195.62 88.38,195.62 J11.8 104.69,195.69 106,194.38 107.61,194.38 108.93,195.69 J1.8 115.31,195.69 116.5,194.5 118.25,194.5 119.38,195.62 120.06,195.62 J2.8 142.19,195.69 151.12,186.75 194.38,186.75 194.5,186.62 211.5,186.62 218,193.12 218,193.25 219,194.25 246.75,194.25 248,195.5 248.63,195.5 J7.8 256.94,195.56 258.25,194.25 260.08,194.25 J12.8
L9
  Top 0.406: X2.15 23.9,167.9 42.75,186.75 51.88,186.75 52,186.62 56.38,186.62 56.5,186.75 58.5,186.75 65,193.25 76.12,193.25 J6.9 76.9,193.15 78.12,194.38 83.75,194.38 84.88,193.25 85.81,193.25 J11.9 86.4,193.15 87.62,194.38 104.75,194.38 106,193.12 107.11,193.12 J1.9 107.65,193.15 109,194.5 115.25,194.5 116.5,193.25 117.49,193.25 J2.9 118.15,193.15 119.5,194.5 140.62,194.5 150.88,184.25 194.5,184.25 194.62,184.12 211.25,184.12 218.75,191.62 218.75,191.88 220,193.12 246.06,193.12 J7.9 246.78,193.03 248.12,194.38 256.88,194.38 258.25,193 258.83,193 J12.9
L10
  Top 0.406: X2.34 23.78,166.53 41.5,184.25 56.5,184.25 56.62,184.12 58.38,184.12 62.12,187.88 62.25,187.88 66.25,191.88 77.11,191.88 78.39,193.15 J6.10 83.72,193.15 85,191.88 86.38,191.88 87.5,193 88.3,193 J11.10 104.72,193.15 106,191.88 108,191.88 109.12,193 109.53,193 J1.10 115.47,193.15 116.75,191.88 118.12,191.88 119.38,193.12 120.11,193.12 J2.10 139.35,193.15 150.75,181.75 194.38,181.75 194.62,181.5 211,181.5 221.25,191.75 246.75,191.75 248.03,193.03 J7.10 256.98,193.03 258.25,191.75 260.12,191.75 J12.10
L11
  Top 0.406: X2.16 23.91,165.16 39.75,181 40.01,181 40.75,181.74 56.5,181.62 57.38,181.62 66.25,190.5 76.11,190.5 J6.11 76.98,190.61 78.25,191.88 83.62,191.88 84.88,190.62 85.89,190.62 J11.11 86.36,190.61 87.5,191.75 104.75,191.75 106,190.5 107.03,190.5 J1.11 107.86,190.61 109,191.75 115.5,191.75 116.62,190.62 117.58,190.62 J2.11 118.11,190.61 119.25,191.75 138,191.75 150.62,179.12 194,179.12 194.12,179 211.5,179 223,190.5 246.15,190.5 J7.11 246.86,190.49 248.25,191.88 257,191.88 258.12,190.75 258.6,190.75 J12.11
L12
  Top 0.406: X2.35 24.14,163.76 39.62,179.25 56.62,179.12 66.88,189.38 76.91,189.38 78.14,190.61 J6.12 83.77,190.61 85,189.38 86.38,189.38 87.5,190.5 88.33,190.5 J11.12 104.39,190.61 105.75,189.25 107.62,189.25 108.88,190.5 109.57,190.5 J1.12 115.39,190.61 116.62,189.38 118.12,189.38 119.25,190.5 120.02,190.5 J2.12 136.64,190.61 150.62,176.62 194.5,176.62 194.62,176.5 211.25,176.5 224,189.25 247.12,189.25 248.36,190.49 J7.12 256.89,190.49 258.12,189.25 259.5,189.25 260.75,190.5 261.38,190.5 J12.12
L13
  Top 0.406: X2.17 24.52,162.39 38.75,176.62 56.5,176.5 68.12,188.12 72.8,188.12 J6.13 76.69,188.07 78,189.38 83.88,189.38 85.12,188.12 85.85,188.12 J11.13 86.32,188.07 87.62,189.38 104.38,189.38 105.62,188.12 107.08,188.12 J1.13 107.69,188.07 109,189.38 115.5,189.38 116.75,188.12 117.53,188.12 J2.13 118.19,188.07 119.5,189.38 136,189.38 151.38,174 211.62,174 225.62,188 246.1,188 J7.13 246.94,187.94 248.25,189.25 256.88,189.25 258.12,188 258.81,188 J12.13
L14
  Top 0.406: X2.36 25.02,161.02 38.12,174.12 52,174.12 52.12,174 56.38,174 69.12,186.75 76.82,186.75 78.14,188.07 J6.14 83.93,188.07 85.25,186.75 86.38,186.75 87.62,188 88.38,188 J11.14 104.43,188.07 105.75,186.75 107.75,186.75 108.88,187.88 109.48,187.88 J1.14 115.43,188.07 116.75,186.75 118.12,186.75 119.38,188 120.06,188 J2.14 134.31,188.07 150.88,171.5 207.25,171.5 207.38,171.38 211.25,171.38 226.5,186.62 246.88,186.62 248.12,187.88 248.63,187.88 J7.14 256.93,187.94 258.25,186.62 259.38,186.62 260.62,187.88 261.33,187.88 J12.14
L15
  Top 0.406: X2.18 25.12,159.62 37,171.5 56.12,171.38 70.25,185.5 72.82,185.5 J6.15 76.66,185.53 77.88,186.75 84,186.75 85.12,185.62 85.81,185.62 J11.15 86.53,185.53 87.75,186.75 104.5,186.75 105.62,185.62 107.05,185.62 J1.15 107.66,185.53 108.88,186.75 115.38,186.75 116.62,185.5 117.56,185.5 J2.15 118.28,185.53 119.5,186.75 133.38,186.75 151.12,169 194.5,169 194.62,168.88 211.5,168.88 228.12,185.5 246.06,185.5 J7.15 246.78,185.41 248,186.62 257.12,186.62 258.25,185.5 258.76,185.5 J12.15
L16
  Top 0.406: X2.37 25.25,158.25 36,169 56.12,168.88 57.62,170.38 57.5,170.5 57.5,171.25 70.5,184.25 76.75,184.25 78.02,185.51 J6.16 83.84,185.53 85.12,184.25 86.5,184.25 87.75,185.5 88.42,185.5 J11.16 104.47,185.53 105.75,184.25 107.75,184.25 108.88,185.38 109.53,185.38 J1.16 115.59,185.53 116.88,184.25 118.12,184.25 119.38,185.5 120.1,185.5 J2.16 131.97,185.53 151,166.5 194.5,166.5 194.62,166.38 211.25,166.38 229,184.12 246.62,184.12 247.88,185.38 248.67,185.38 J7.16 256.72,185.41 258,184.12 260.12,184.12 J12.16
L17
  Top 0.406: X3.11 22,107.83 24.04,109.88 24.12,109.88 27,112.75 27,151.88 41.5,166.38 56.88,166.38 58.75,168.25 58.75,170.38 71.36,182.99 J6.17 76.61,182.99 77.88,184.25 83.75,184.25 85,183 85.89,183 | 85.89,183 J11.17 | 85.89,183 86.5,183 87.75,184.25 104.5,184.25 105.62,183.12 107,183.12 J1.17 107.61,182.99 108.88,184.25 115.75,184.25 116.88,183.12 117.45,183.12 J2.17 118.11,182.99 119.38,184.25 130.25,184.25 150.62,163.88 194.5,163.88 194.62,163.75 211.5,163.75 230.75,183 246.03,183 J7.17 246.74,182.87 248,184.12 256.62,184.12 257.88,182.88 J12.17
L18
  Top 0.406: X3.30 21.02,106.38 22.25,106.38 28.38,112.5 28.38,151 41.25,163.88 56.75,163.88 59.62,166.75 59.62,166.88 61.62,168.88 61.62,170.25 70.38,179 70.38,179.12 73,181.75 76.88,181.75 78.02,182.89 J6.18 83.64,182.99 84.88,181.75 86.5,181.75 87.62,182.88 88.33,182.88 J11.18 104.39,182.99 105.62,181.75 107.75,181.75 108.88,182.88 109.56,182.88 J1.18 115.64,182.99 116.88,181.75 118.12,181.75 119.25,182.88 120.02,182.88 J2.18 120.37,182.75 129.75,182.75 151.12,161.38 194.5,161.38 194.62,161.25 211.62,161.25 232,181.62 246.88,181.62 248,182.75 248.59,182.75 J7.18 256.38,182.87 257.62,181.62 259.5,181.62 260.62,182.75 261.29,182.75 J12.18
L19
  Top 0.406: X3.12 18.12,105.12 22.88,105.12 29.5,111.75 29.5,150.38 40.25,161.12 56.5,161.12 62.75,167.38 62.75,170.12 72,179.38 72,179.45 73,180.45 J6.19 76.7,180.45 78,181.75 83.75,181.75 85,180.5 85.86,180.5 J11.19 86.45,180.45 87.75,181.75 104.25,181.75 105.62,180.38 107.06,180.38 J1.19 107.83,180.45 109.12,181.75 115.62,181.75 116.88,180.5 117.54,180.5 J2.19 118.2,180.45 119.5,181.75 128.12,181.75 151,158.88 194.62,158.88 194.75,158.75 212.12,158.75 233.62,180.25 246.09,180.25 J7.19 246.82,180.32 248,181.5 256.38,181.5 257.62,180.25 258.79,180.25 J12.19
L20
  Top 0.406: X3.31 21.12,103.88 23.12,103.88 30.75,111.5 30.75,149.62 41.12,160 57.25,160 63.5,166.25 63.5,169.75 73,179.25 76.88,179.25 78.08,180.45 J6.20 83.55,180.45 84.88,179.12 86.5,179.12 87.75,180.38 88.37,180.38 J11.20 104.05,180.45 105.38,179.12 108,179.12 109.12,180.25 109.48,180.25 J1.20 115.55,180.45 116.75,179.25 118.25,179.25 119.38,180.38 120.06,180.38 J2.20 120.18,180.5 128.25,180.5 150.62,158.12 192.75,158.12 194.62,156.25 212,156.25 234.25,178.5 234.38,178.5 234.88,179 246.75,179 248.07,180.32 J7.20 256.05,180.32 257.38,179 260.07,179 J12.20
L21
  Top 0.406: X3.13 18.16,102.25 23.25,102.25 64.5,143.5 64.5,169.38 73.03,177.91 J6.21 76.78,177.91 78.12,179.25 83.5,179.25 84.88,177.88 85.87,177.88 J11.21 86.53,177.91 87.88,179.25 104,179.25 105.38,177.88 107.11,177.88 J1.21 107.91,177.91 109.25,179.25 115.62,179.25 116.88,178 117.5,178 J2.21 118.16,177.91 119.5,179.25 128.25,179.25 128.38,179.12 128.5,179.12 150.38,157.25 190.25,157.25 194.12,153.38 211.38,153.38 235.62,177.62 246,177.62 J7.21 246.91,177.78 248.12,179 255.75,179 257,177.75 258.82,177.75 J12.21
L22
  Top 0.406: X3.32 21.14,101.12 23.88,101.12 65.25,142.5 65.25,169 73,176.75 77,176.75 78.16,177.91 J6.22 83.72,177.91 85,176.62 86.38,176.62 87.62,177.88 88.41,177.88 J11.22 103.84,177.91 105.12,176.62 107.75,176.62 108.88,177.75 109.52,177.75 J1.22 115.34,177.91 116.5,176.75 118.12,176.75 119.25,177.88 120.09,177.88 J2.22 120.17,177.88 128.38,177.88 136.12,170.12 136.25,170.12 150,156.38 189.88,156.38 193.62,152.62 212.25,152.62 236.12,176.5 246.88,176.5 248.07,177.7 J7.22 255.72,177.78 257,176.5 260.12,176.5 J12.22
L23
  Top 0.406: X3.14 18.16,99.62 23.75,99.62 23.88,99.75 24,99.75 66.12,141.88 66.12,168.62 72.87,175.37 J6.23 76.87,175.37 78.12,176.62 83.75,176.62 85,175.38 J11.23 86.37,175.37 87.62,176.62 104,176.62 105.25,175.38 J1.23 107.62,175.37 109,176.75 115.25,176.75 116.62,175.38 J2.23 118.12,175.37 119.5,176.75 128.25,176.75 149.62,155.38 189.75,155.38 193.25,151.88 213.12,151.88 236.62,175.38 245.25,175.38 245.62,175 245.91,175 J7.23 246.75,175.25 248,176.5 255.62,176.5 256.88,175.25 J12.23
L24
  Top 0.406: X3.33 21,98.25 23.75,98.25 67,141.5 67,168.5 72.62,174.12 77.25,174.12 78.5,175.37 J6.24 83.88,175.37 85.12,174.12 86.5,174.12 87.62,175.25 88.33,175.25 J11.24 104,175.37 105.25,174.12 107.62,174.12 108.88,175.38 J1.24 115.38,175.37 116.62,174.12 118.12,174.12 119.38,175.38 J2.24 128.62,175.38 149.38,154.62 189.12,154.62 192.75,151 213.75,151 236.75,174 246.62,174 247.88,175.25 J7.24 255.5,175.25 256.75,174 260.15,174 J12.24
L25
  Top 0.406: X3.15 18.18,96.88 23.5,96.88 67.88,141.25 67.88,168.12 72.58,172.83 J6.25 77.08,172.83 78.38,174.12 83.88,174.12 85.12,172.88 85.86,172.88 J11.25 86.33,172.83 87.62,174.12 103.88,174.12 105.12,172.88 107.09,172.88 J1.25 107.58,172.83 108.88,174.12 115.38,174.12 116.62,172.88 117.55,172.88 J2.25 118.08,172.83 119.38,174.12 128.88,174.12 149.12,153.88 188.88,153.88 192.5,150.25 214.5,150.25 237,172.75 246.12,172.75 J7.25 246.83,172.71 248,173.88 255.62,173.88 256.88,172.62 258.78,172.62 J12.25
L26
  Top 0.406: X3.34 21.02,95.5 23.38,95.5 41.31,113.44 41.5,113.62 68.62,140.75 68.62,167.62 72.62,171.62 77.12,171.62 78.27,172.76 J6.26 83.8,172.83 85,171.62 86.75,171.62 87.88,172.75 88.36,172.75 J11.26 103.92,172.83 105.12,171.62 107.75,171.62 108.88,172.75 109.6,172.75 J1.26 115.42,172.83 116.62,171.62 118.12,171.62 119.25,172.75 120.05,172.75 J2.26 120.17,172.88 129,172.88 148.75,153.12 188.25,153.12 192,149.38 214.88,149.38 237,171.5 247,171.5 248.25,172.75 248.66,172.75 J7.26 255.54,172.71 256.75,171.5 260.19,171.5 J12.26
L27
  Top 0.406: X3.16 18.13,94 23.62,94 41.81,112.19 42.5,112.88 69.5,139.88 69.5,167.38 72.42,170.29 J6.27 76.92,170.29 78.25,171.62 83.75,171.62 85,170.38 85.82,170.38 J11.27 86.54,170.29 87.88,171.62 103.75,171.62 105.12,170.25 107.1,170.25 J1.27 107.67,170.29 108.88,171.5 115.62,171.5 116.75,170.38 117.5,170.38 J2.27 118.04,170.29 119.38,171.62 119.5,171.5 129.12,171.5 151.62,149 187.25,149 193.12,143.12 212.88,143.12 239.88,170.12 246.12,170.12 J7.27 | 246,170 J7.27 | J7.27 246.91,170.16 248.12,171.38 255.25,171.38 256.5,170.12 258.82,170.12 J12.27
L28
  Top 0.406: X3.35 21.16,92.88 23.88,92.88 70.38,139.38 70.38,166.88 72.5,169 76.88,169 78.14,170.26 J6.28 83.96,170.29 85.25,169 86.5,169 87.62,170.12 88.28,170.12 J11.28 103.83,170.29 105.12,169 107.75,169 109,170.25 109.64,170.25 J1.28 115.58,170.29 116.88,169 118.12,169 119.38,170.25 120.09,170.25 J2.28 120.3,170.12 129.38,170.12 151.25,148.25 186.62,148.25 192.62,142.25 213.38,142.25 215.75,144.62 215.75,144.75 239.5,168.5 239.62,168.5 240,168.88 246.88,168.88 248.12,170.12 248.66,170.12 J7.28 255.34,170.16 256.62,168.88 260.11,168.88 J12.28
L29
  Top 0.406: X3.17 18.11,91.25 23.38,91.25 44.38,112.25 44.5,112.25 59.25,127 59.25,127.25 71,139 71,153.62 71.12,153.75 71.12,166.5 72.38,167.75 J6.29 76.88,167.75 78.12,169 83.75,169 85,167.75 J11.29 86.5,167.75 87.75,169 103.88,169 105.12,167.75 J1.29 107.75,167.75 109,169 115.5,169 116.75,167.75 J2.29 118.12,167.75 119.38,169 129.25,169 150.75,147.5 186.12,147.5 192.12,141.5 213.75,141.5 239.75,167.5 246.03,167.5 J7.29 246.75,167.62 248,168.88 255.25,168.88 256.62,167.5 258.74,167.5 J12.29
L30
  Top 0.406: X3.36 21.03,90 23.38,90 45.5,112.12 45.88,112.12 71.75,138 71.75,153 71.88,153.12 71.88,165.75 72.62,166.5 76.88,166.5 78.12,167.75 J6.30 83.5,167.75 84.75,166.5 86.38,166.5 87.5,167.62 88.32,167.62 J11.30 104,167.75 105.25,166.5 107.88,166.5 109.12,167.75 J1.30 115.5,167.75 116.75,166.5 118,166.5 119.25,167.75 J2.30 129.25,167.75 150.25,146.75 185.62,146.75 191.62,140.75 214.25,140.75 239.88,166.38 246.88,166.38 248,167.5 248.57,167.5 J7.30 255.12,167.62 256.38,166.38 260.15,166.38 J12.30
L31
  Top 0.406: X3.18 18.21,88.62 23.25,88.62 46.38,111.75 46.5,111.75 72.5,137.75 72.5,152.5 72.44,152.56 72.62,152.75 72.62,164.75 73.08,165.21 J6.31 76.83,165.21 78.12,166.5 83.75,166.5 85,165.25 85.86,165.25 J11.31 86.46,165.21 87.75,166.5 104,166.5 105.12,165.38 106.97,165.38 J1.31 107.96,165.21 109.25,166.5 115.38,166.5 116.62,165.25 117.55,165.25 J2.31 118.08,165.21 119.38,166.5 129.38,166.5 149.88,146 185.25,146 191.25,140 214.62,140 239.62,165 246.07,165 J7.31 246.84,165.09 248.12,166.38 255.12,166.38 256.38,165.12 258.82,165.12 J12.31
L32
  Top 0.406: X3.37 21.3,87.5 23.38,87.5 73.12,137.25 73.12,152.12 73.5,152.5 73.5,163.12 74.38,164 77.12,164 78.14,165.01 78.77,165.01 J6.32 83.79,165.21 85.12,163.88 86.38,163.88 87.62,165.12 88.36,165.12 J11.32 103.79,165.21 105.12,163.88 107.62,163.88 108.88,165.12 109.59,165.12 J1.32 115.54,165.21 116.88,163.88 118.25,163.88 119.5,165.12 120.05,165.12 J2.32 129.29,165.21 149.38,145.12 184.75,145.12 190.62,139.25 215.12,139.25 239.62,163.75 246.88,163.75 248.12,165 248.62,165 J7.32 254.79,165.09 256.12,163.75 260.06,163.75 J12.32
L33
  Top 0.406: X4.11 18.15,35.38 22.25,35.38 48.25,61.38 48.25,61.75 74,87.5 74,151.75 74.25,152 74.25,161.38 75.55,162.67 J6.33 77.05,162.67 78.25,163.88 84,163.88 85.25,162.62 85.86,162.62 J11.33 86.42,162.67 87.62,163.88 103.88,163.88 105.12,162.62 107.09,162.62 J1.33 107.8,162.67 109,163.88 115.5,163.88 116.62,162.75 117.51,162.75 J2.33 118.42,162.67 119.62,163.88 129.5,163.88 149.25,144.12 184.38,144.12 190,138.5 216.25,138.5 240.25,162.5 246.12,162.5 J7.33 246.79,162.54 248,163.75 255,163.75 256.12,162.62 258.78,162.62 J12.33
L34
  Top 0.406: X4.30 21,34 22.62,34 49.25,60.62 49.25,60.75 81,92.5 81,162.62 80.95,162.67 J6.34 83.58,162.67 84.88,161.38 87.15,161.38 J11.34 103.83,162.67 105.12,161.38 107.88,161.38 109.12,162.62 109.64,162.62 J1.34 115.33,162.67 116.62,161.38 118.25,161.38 119.38,162.5 119.96,162.5 J2.34 129.33,162.67 148.75,143.25 183.88,143.25 189.62,137.5 216.62,137.5 240.25,161.12 240.38,161.12 240.5,161.25 246.75,161.25 248,162.5 248.66,162.5 J7.34 254.96,162.54 256.25,161.25 260.11,161.25 J12.34
L35
  Top 0.406: J1.35 107.75,160.13 | 107.75,160.13 109.12,161.5 115.25,161.5 116.62,160.12 J2.35 118.5,160.13 119.75,161.38 129.38,161.38 148.38,142.38 183.62,142.38 189.25,136.75 217.25,136.75 240.5,160 J7.35 246.88,160 248,161.12 255.25,161.12 256.38,160 J12.35 | X4.12 18.16,32.62 23.38,32.62 105.25,114.5 105.25,157.62 107.75,160.13
L36
  Top 0.406: J1.36 109.68,158.44 109.75,158.38 117.88,158.38 119.5,160 120,160 J2.36 127.25,160.13 | 127.25,160.13 129.25,160.13 147.88,141.5 183.12,141.5 188.75,135.88 218,135.88 240.75,158.62 246.69,158.62 248.07,160 J7.36 255.12,160 256.5,158.62 260.02,158.62 J12.36 | X4.31 20.98,31.25 23.88,31.25 52.25,59.62 52.25,59.75 95,102.5 95,102.75 127,134.75 127,159.88 127.25,160.13
L37
  Top 0.406: X4.13 18.14,29.88 24.25,29.88 53.62,59.25 53.75,59.25 122.75,128.25 122.75,128.38 129,134.62 218.62,134.62 241.47,157.47 J7.37 246.84,157.47 248,158.62 255.25,158.62 256.38,157.5 258.82,157.5 J12.37
L38
  Top 0.406: X4.32 24.78,28.53 129.75,133.5 219,133.5 241.75,156.25 246.88,156.25 248,157.38 248.61,157.38 J7.38 255.16,157.47 256.5,156.12 259.62,156.12 260.88,157.38 261.31,157.38 J12.38
L39
  Top 0.406: X4.14 24.91,27.16 128.75,131 128.88,131 130,132.12 219,132.12 241.75,154.88 246.11,154.88 J7.39 246.8,154.93 248.12,156.25 255.12,156.25 256.5,154.88 258.81,154.88 J12.39
L40
  Top 0.406: X4.33 21.02,25.88 25.25,25.88 97.62,98.25 97.75,98.25 130.62,131.12 219.5,131.12 241.88,153.5 246.5,153.5 247.93,154.93 J7.40 255.32,154.93 256.62,153.62 259.5,153.62 260.75,154.88 261.35,154.88 J12.40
